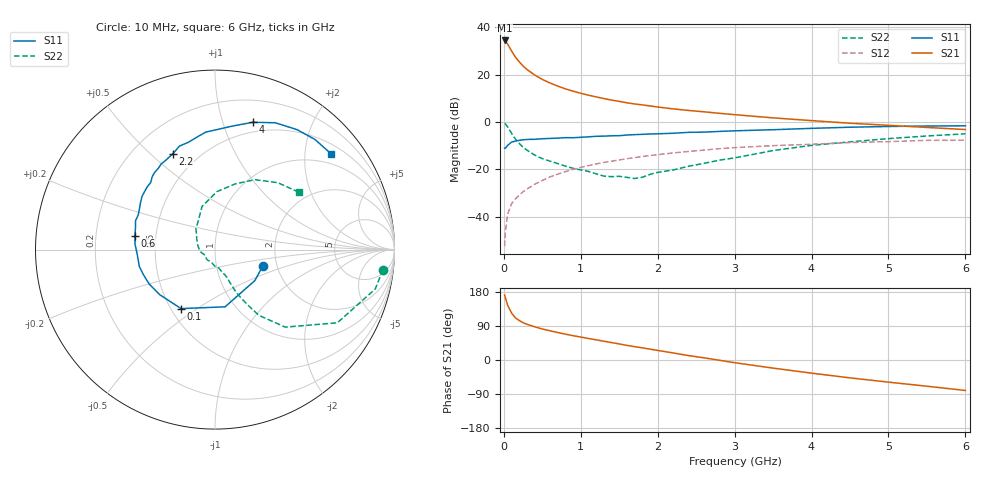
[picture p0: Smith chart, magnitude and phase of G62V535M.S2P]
! SIEMENS Small Signal Semiconductors
! BFG193
! Si NPN RF Bipolar Junction Transistor in SOT223
! VCE = 2.5 V  IC = 35 mA
! Common Emitter S-Parameters:  August  1996
# GHz  S  MA  R  50
!  f  S11  S21  S12  S22
! GHz  MAG  ANG  MAG  ANG  MAG  ANG  MAG  ANG
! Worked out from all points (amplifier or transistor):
!   36 points, 10 MHz to 6 GHz, reference 50 ohm
!   highest |S21| = 34.5 dB at 10 MHz (marker M1)
!   |S21| within 3 dB of that: start of sweep to 75.02 MHz
!   unconditionally stable (mu >= 1): 487.4 MHz to 2.376 GHz
!   at 250 MHz: K = 0.87, MSG = 26.6 dB, |S12| = -29.4 dB
!   at 1.4 GHz: K = 1.05, MAG = 11.6 dB, |S12| = -16.5 dB
!   at 6 GHz: K = 0.91, MSG = 2.2 dB, |S12| = -7.6 dB
!   S11 on the Smith chart (normalised r, x): 10 MHz: 1.68, -0.34; 100 MHz: 0.56, -0.43; 600 MHz: 0.38, +0.07; 2.2 GHz: 0.36, +0.59; 4 GHz: 0.40, +1.26; 6 GHz: 0.73, +2.61
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0.01  0.281 -19.4  53.23 171.6  0.0024 87.9  0.9424 -6.8
0.02  0.2814 -37.7  51.58 164.3  0.0049 78.5  0.9195 -13.8
0.05  0.3238 -80.0  44.27 144.0  0.0114 70.4  0.7943 -30.9
0.1  0.3791 -119.9  32.08 124.1  0.0189 64.1  0.583 -47.8
0.15  0.3977 -140.9  23.74 111.3  0.0239 62.5  0.4401 -56.3
0.2  0.4135 -152.3  18.82 104.2  0.0287 64.5  0.3562 -59.5
0.25  0.4229 -160.9  15.38 98.4  0.0338 64.7  0.2935 -62.3
0.3  0.432 -167.5  13.01 94.2  0.0388 65.7  0.2569 -63.9
0.4  0.4342 -176.6  9.94 87.8  0.0487 66.5  0.2021 -65.6
0.5  0.4469 175.9  7.99 81.8  0.0587 65.4  0.1695 -66.6
0.6  0.4528 170.2  6.721 77.1  0.0696 64.8  0.1502 -68.8
0.7  0.4597 164.4  5.783 72.5  0.0797 63.8  0.1337 -72.2
0.8  0.4712 160.1  5.055 68.2  0.09 61.9  0.1179 -75.3
1.1  0.49 148.0  3.711 56.8  0.1207 57.1  0.091 -91.4
1.6  0.5358 130.8  2.565 38.6  0.1693 46.3  0.0683 -137.0
2.2  0.5827 113.9  1.907 18.6  0.2237 32.7  0.0975 167.3
2.8  0.6374 98.5  1.539 -0.6  0.2748 18.7  0.1572 132.5
3.5  0.6927 82.5  1.233 -21.4  0.3189 1.4  0.2514 106.6
4  0.7399 73.5  1.078 -34.7  0.3415 -8.4  0.3232 88.1
4.5  0.7823 64.6  0.949 -47.2  0.3705 -18.5  0.3835 72.8
5.5  0.8287 47.8  0.774 -69.2  0.4128 -41.6  0.5112 46.8
6  0.8387 39.4  0.698 -80.4  0.4171 -54.9  0.5669 34.3
